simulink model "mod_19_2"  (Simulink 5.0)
settings: Solver=ode1  StartTime=0.0  StopTime=200  FixedStep=0.002  MaxStep=0.01  MinStep=0.0001  RelTol=1e-3
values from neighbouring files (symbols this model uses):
  Acp = 5.249    [dados_19_2.m]
  Apr = 5.249    [dados_19_2.m]
  CA0 = 12.815    [dados_19_2.m]
  CB0 = 0    [dados_19_2.m]
  cp = 0.12    [dados_19_2.m]
  cPa = 1.0    (= 1)    [dados_19_2.m]
  cPr = 1.0    (= 1)    [dados_19_2.m]
  Cva = 100    [dados_19_2.m]
  Cvv = 1.65    [dados_19_2.m]
  dPa = 1.406    [dados_19_2.m]
  G = 0.99803    [dados_19_2.m]
  hv_tab = [2706.3 2708.5 2710.6 2712.6 2714.5 2716.4 2718.2 2719.9 2721.5 2723.1 2724.7            2726.1 2727.6 2729.0 2730.0 2731.6]*0.2388459    [dados_19_2.m]
  k10 = 729.55    [dados_19_2.m]
  k20 = 6567.6    [dados_19_2.m]
  Kc = 2    [dados_19_2.m]
  Km = (Tmed_max-Tmed_min)/(Tmax-Tmin)    (= 0.109090909091)    [dados_19_2.m]
  Kva = 0.014276    [dados_19_2.m]
  Kvv = 6.4516    [dados_19_2.m]
  Lambda1 = 22222    [dados_19_2.m]
  Lambda2 = 27778    [dados_19_2.m]
  mcbarra = 7    [dados_19_2.m]
  Pv0 = 2.419    [dados_19_2.m]
  Pv_alim = 2.461    [dados_19_2.m]
  Pv_tab = [   2.0    2.1    2.2    2.3    2.4    2.5    2.6    2.7    2.8    2.9    3.0               3.1    3.2    3.3    3.4    3.5]*1.019716    [dados_19_2.m]
  R = 1.9858    [dados_19_2.m]
  rampa = 0.005    [dados_19_2.m]
  rho = 800.92    [dados_19_2.m]
  rhoa = 997.048    [dados_19_2.m]
  rhop = 8201.5    [dados_19_2.m]
  rhov_tab = [1/0.8854 1/0.8459 1/0.8098 1/0.7768 1/0.7465 1/0.7184 1/0.6925 1/0.6684 1/0.6460            1/0.6251 1/0.6056 1/0.5872 1/0.5700 1/0.5538 1/0.5385 1/0.5240]    [dados_19_2.m]
  T0 = 25    [dados_19_2.m]
  Tae = 25    [dados_19_2.m]
  talm = 4/60    (= 0.0666666666667)    [dados_19_2.m]
  Tlim = 93    [dados_19_2.m]
  Tmed0 = Km*(T0-Tmin)+Tmed_min    (= 4.63636363636)    [dados_19_2.m]
  Tmed_max = 15    [dados_19_2.m]
  Tmed_min = 3    [dados_19_2.m]
  Tmin = 10    [dados_19_2.m]
  Tp0 = 25    [dados_19_2.m]
  Tref0 = 12.6    [dados_19_2.m]
  Tv_tab = [120.23 121.78 123.27 124.71 126.09 127.43 128.73 129.98 131.20 132.39 133.54            134.66 135.75 136.82 137.86 138.87]    [dados_19_2.m]
  Uap = 32.550    (= 32.55)    [dados_19_2.m]
  Upr = 13.020    (= 13.02)    [dados_19_2.m]
  Uvp = 81.374    [dados_19_2.m]
  V = 1.2035    [dados_19_2.m]
  Vcam = 0.5332    [dados_19_2.m]
  Vp = 0.2667    [dados_19_2.m]
  xT = 0.75    [dados_19_2.m]
libraries: simulink_extras x1

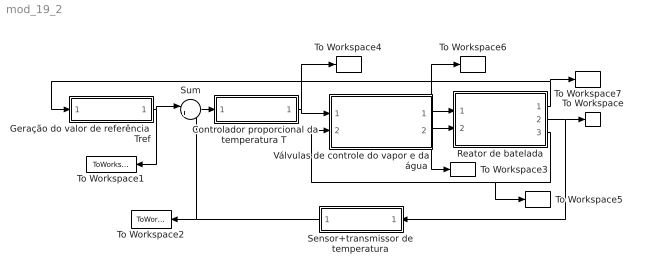
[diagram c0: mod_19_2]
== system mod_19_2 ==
  "Controlador proporcional da temperatura T " : Subsystem
  Geração do valor de referência Tref : Subsystem
  Reator de batelada : Subsystem
  Sensor+transmissor de temperatura : Subsystem  Orientation=left
  Sum : Sum  Inputs=|+-
  To Workspace : ToWorkspace  VariableName=T  SampleTime=-1  SaveFormat=Array
  To Workspace1 : ToWorkspace  VariableName=Tref_psi  SampleTime=-1  SaveFormat=Array
  To Workspace2 : ToWorkspace  VariableName=Tmed  SampleTime=-1  SaveFormat=Array
  To Workspace3 : ToWorkspace  VariableName=Wv  SampleTime=-1  SaveFormat=Array
  To Workspace4 : ToWorkspace  VariableName=mc  SampleTime=-1  SaveFormat=Array
  To Workspace5 : ToWorkspace  VariableName=Pv  SampleTime=-1  SaveFormat=Array
  To Workspace6 : ToWorkspace  VariableName=Qa  SampleTime=-1  SaveFormat=Array
  To Workspace7 : ToWorkspace  VariableName=Chav  SampleTime=-1  SaveFormat=Array
  "Válvulas de controle do vapor e da água " : Subsystem
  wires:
  Reator de batelada/1(Chav) -> Geração do valor de referência Tref/1(Chav), To Workspace7/1
  "Válvulas de controle do vapor e da água "/1(Qa) -> To Workspace6/1, Reator de batelada/1(Qa)
  "Controlador proporcional da temperatura T "/1(mc) -> To Workspace4/1, "Válvulas de controle do vapor e da água "/1(mc)
  Sum/1 -> "Controlador proporcional da temperatura T "/1(ec)
  Geração do valor de referência Tref/1(Tref_psi) -> Sum/1, To Workspace1/1
  Sensor+transmissor de temperatura/1(Tmed) -> Sum/2, To Workspace2/1
  Reator de batelada/2(T) -> To Workspace/1, Sensor+transmissor de temperatura/1(T)
  Reator de batelada/3(Pv) -> "Válvulas de controle do vapor e da água "/2(Pv), To Workspace5/1
  "Válvulas de controle do vapor e da água "/2(Wv) -> To Workspace3/1, Reator de batelada/2(Wv)

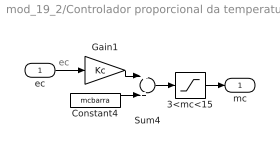
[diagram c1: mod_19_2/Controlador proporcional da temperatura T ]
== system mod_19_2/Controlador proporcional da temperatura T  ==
  note: ec
  ec : Inport
  3<mc<15 : Saturate  UpperLimit=15  LowerLimit=3
  Constant4 : Constant  Value=mcbarra
  Gain1 : Gain  Gain=Kc
  Sum4 : Sum  Inputs=2
  mc : Outport
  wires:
  ec/1 -> Gain1/1
  Gain1/1 -> Sum4/1
  Constant4/1 -> Sum4/2
  Sum4/1 -> 3<mc<15/1
  3<mc<15/1 -> mc/1

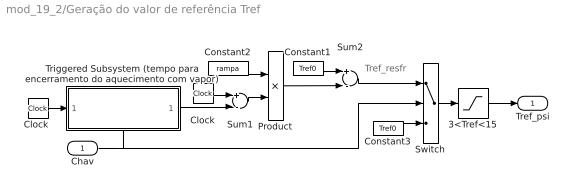
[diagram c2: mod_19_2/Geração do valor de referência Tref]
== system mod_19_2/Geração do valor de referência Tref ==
  note: Tref_resfr
  Chav : Inport
  3<Tref<15 : Saturate  UpperLimit=Tmed_max  LowerLimit=Tmed_min
  Clock : Clock
  "Clock " : Clock
  Constant1 : Constant  Value=Tref0
  Constant2 : Constant  Value=rampa
  Constant3 : Constant  Value=Tref0
  Product : Product
  Sum1 : Sum  Inputs=+-
  Sum2 : Sum  Inputs=+-
  Switch : Switch  Threshold=0.5
  Triggered Subsystem (tempo para encerramento do aquecimento com vapor) : Subsystem  TreatAsAtomicUnit=on
  Tref_psi : Outport
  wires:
  Triggered Subsystem (tempo para encerramento do aquecimento com vapor)/1(t_inicio_resfr) -> Sum1/2
  Constant3/1 -> Switch/3
  Switch/1 -> 3<Tref<15/1
  Sum2/1 -> Switch/1
  "Clock "/1 -> Triggered Subsystem (tempo para encerramento do aquecimento com vapor)/1(tempo)
  Chav/1 -> Triggered Subsystem (tempo para encerramento do aquecimento com vapor)/Trigger, Switch/2
  Clock/1 -> Sum1/1
  Sum1/1 -> Product/2
  Constant2/1 -> Product/1
  Constant1/1 -> Sum2/1
  Product/1 -> Sum2/2
  3<Tref<15/1 -> Tref_psi/1

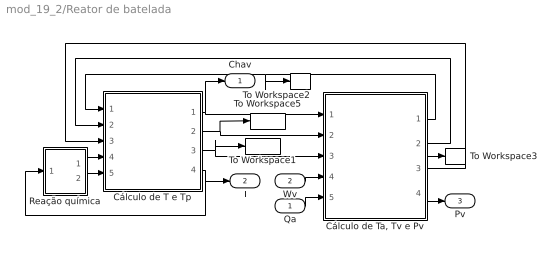
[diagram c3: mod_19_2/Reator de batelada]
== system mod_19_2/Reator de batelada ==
  Qa : Inport
  Wv : Inport  Port=2
  Cálculo de T e Tp : Subsystem
  "Cálculo de Ta, Tv e Pv" : Subsystem
  Reação química : Subsystem
  To Workspace1 : ToWorkspace  VariableName=qcp_r  SampleTime=-1  SaveFormat=Array
  To Workspace2 : ToWorkspace  VariableName=Tv  SampleTime=-1  SaveFormat=Array
  To Workspace3 : ToWorkspace  VariableName=Ta  SampleTime=-1  SaveFormat=Array
  To Workspace5 : ToWorkspace  VariableName=qcp_a  SampleTime=-1  SaveFormat=Array
  Chav : Outport
  T : Outport  Port=2
  Pv : Outport  Port=3
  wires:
  Qa/1 -> "Cálculo de Ta, Tv e Pv"/5(Qa)
  Wv/1 -> "Cálculo de Ta, Tv e Pv"/4(Wv)
  "Cálculo de Ta, Tv e Pv"/4(Pv) -> Pv/1
  Cálculo de T e Tp/2(qcp_aquec) -> "Cálculo de Ta, Tv e Pv"/2(qcp_aquec), To Workspace5/1
  "Cálculo de Ta, Tv e Pv"/1(Tv) -> Cálculo de T e Tp/1(Tv), To Workspace2/1
  Cálculo de T e Tp/1(Chav) -> "Cálculo de Ta, Tv e Pv"/1(Chav), Chav/1
  Cálculo de T e Tp/4(T) -> Reação química/1(T), T/1
  Reação química/2(q2) -> Cálculo de T e Tp/5(q2)
  Reação química/1(q1) -> Cálculo de T e Tp/4(q1)
  "Cálculo de Ta, Tv e Pv"/2(Ta) -> Cálculo de T e Tp/2(Ta), To Workspace3/1
  "Cálculo de Ta, Tv e Pv"/3(Va,cam) -> Cálculo de T e Tp/3(Va,cam)
  Cálculo de T e Tp/3(qcp_resfr) -> "Cálculo de Ta, Tv e Pv"/3(qcp_resfr), To Workspace1/1

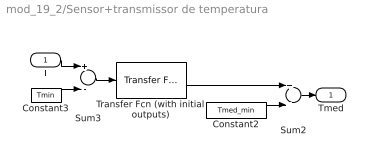
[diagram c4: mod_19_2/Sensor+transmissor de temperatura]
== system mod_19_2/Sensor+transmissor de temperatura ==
  T : Inport
  Constant2 : Constant  Value=Tmed_min
  Constant3 : Constant  Value=Tmin
  Sum2 : Sum  Inputs=2
  Sum3 : Sum  Inputs=+-
  Transfer Fcn (with initial outputs) : simulink_extras/Additional Linear/Transfer Fcn (with initial outputs)  N=[Km]  D="[talm  1]"  Y0=Tmed0-Tmed_min  U0=0
  Tmed : Outport
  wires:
  T/1 -> Sum3/1
  Sum2/1 -> Tmed/1
  Constant3/1 -> Sum3/2
  Sum3/1 -> Transfer Fcn (with initial outputs)/1
  Transfer Fcn (with initial outputs)/1 -> Sum2/1
  Constant2/1 -> Sum2/2

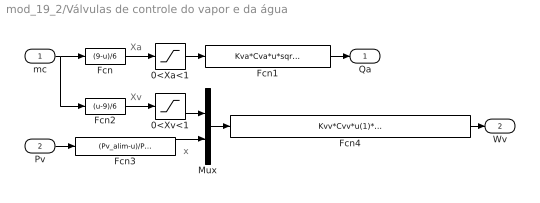
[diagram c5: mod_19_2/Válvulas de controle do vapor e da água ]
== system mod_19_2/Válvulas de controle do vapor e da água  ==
  note: Xa
  note: Xv
  note: x
  mc : Inport
  Pv : Inport  Port=2
  0<Xa<1 : Saturate  UpperLimit=1  LowerLimit=0
  0<Xv<1 : Saturate  UpperLimit=1  LowerLimit=0
  Fcn : Fcn  Expr=(9-u)/6
  Fcn1 : Fcn  Expr=Kva*Cva*u*sqrt(dPa/G)
  Fcn2 : Fcn  Expr=(u-9)/6
  Fcn3 : Fcn  Expr=(Pv_alim-u)/Pv_alim
  Fcn4 : Fcn  Expr=Kvv*Cvv*u(1)*Pv_alim*(3-u(2)/xT)*sqrt(u(2))
  Mux : Mux  Inputs=2
  Qa : Outport
  Wv : Outport  Port=2
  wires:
  mc/1 -> Fcn/1, Fcn2/1
  Fcn/1 -> 0<Xa<1/1
  0<Xa<1/1 -> Fcn1/1
  Fcn2/1 -> 0<Xv<1/1
  0<Xv<1/1 -> Mux/1
  Fcn1/1 -> Qa/1
  Pv/1 -> Fcn3/1
  Mux/1 -> Fcn4/1
  Fcn4/1 -> Wv/1
  Fcn3/1 -> Mux/2

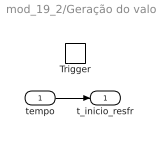
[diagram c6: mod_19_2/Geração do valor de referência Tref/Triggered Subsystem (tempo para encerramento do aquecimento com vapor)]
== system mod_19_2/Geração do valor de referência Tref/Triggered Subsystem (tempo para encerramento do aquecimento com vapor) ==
  tempo : Inport
  Trigger : TriggerPort
  t_inicio_resfr : Outport
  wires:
  tempo/1 -> t_inicio_resfr/1

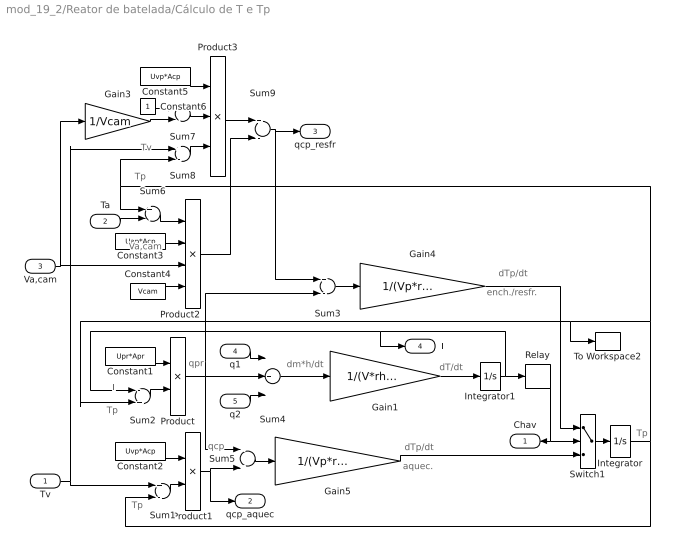
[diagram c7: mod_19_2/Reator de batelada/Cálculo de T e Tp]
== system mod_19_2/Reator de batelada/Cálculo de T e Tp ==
  note: Tp
  note: dTp/dt
  note: T
  note: dT/dt
  note: dm*h/dt
  note: qcp
  note: Tp
  note: qpr
  note: Tp
  note: aquec.
  note: Va,cam
  note: Tp
  note: Tv
  note: dTp/dt
  note: ench./resfr.
  Tv : Inport
  Ta : Inport  Port=2
  Va,cam : Inport  Port=3
  q1 : Inport  Port=4
  q2 : Inport  Port=5
  Constant1 : Constant  Value=Upr*Apr
  Constant2 : Constant  Value=Uvp*Acp
  Constant3 : Constant  Value=Uap*Acp
  Constant4 : Constant  Value=Vcam
  Constant5 : Constant  Value=Uvp*Acp
  Constant6 : Constant
  Gain1 : Gain  Gain=1/(V*rho*cPr)
  Gain3 : Gain  Gain=1/Vcam
  Gain4 : Gain  Gain=1/(Vp*rhop*cp)
  Gain5 : Gain  Gain=1/(Vp*rhop*cp)
  Integrator : Integrator  InitialCondition=Tp0
  Integrator1 : Integrator  InitialCondition=T0
  Product : Product
  Product1 : Product
  Product2 : Product  Inputs=***/
  Product3 : Product  Inputs=3
  Relay : Relay  OnSwitchValue=Tlim  OffSwitchValue=T0
  Sum{1,3,6..9} (6 alike) : Sum  Inputs=+-
  Sum2 : Sum  Inputs=-+
  Sum4 : Sum  Inputs=3
  Sum5 : Sum  Inputs=-+
  Switch1 : Switch  Threshold=0.5
  To Workspace2 : ToWorkspace  VariableName=Tp  SampleTime=-1  SaveFormat=Array
  Chav : Outport  Orientation=left
  qcp_aquec : Outport  Port=2
  qcp_resfr : Outport  Port=3
  T : Outport  Port=4
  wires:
  Integrator1/1 -> Relay/1, Sum2/1, T/1
  Integrator/1 -> Sum1/2, Sum2/2, To Workspace2/1, Sum6/1, Sum8/2
  Sum1/1 -> Product1/2
  Gain1/1 -> Integrator1/1
  Sum4/1 -> Gain1/1
  q1/1 -> Sum4/1
  q2/1 -> Sum4/3
  Product1/1 -> qcp_aquec/1, Sum5/2
  Tv/1 -> Sum1/1, Sum8/1
  Product/1 -> Sum5/1, Sum4/2, Sum3/2
  Constant1/1 -> Product/1
  Sum2/1 -> Product/2
  Constant2/1 -> Product1/1
  Constant3/1 -> Product2/2
  Va,cam/1 -> Product2/3, Gain3/1
  Constant4/1 -> Product2/4
  Ta/1 -> Sum6/2
  Sum6/1 -> Product2/1
  Gain3/1 -> Sum7/2
  Constant6/1 -> Sum7/1
  Sum7/1 -> Product3/2
  Constant5/1 -> Product3/1
  Sum8/1 -> Product3/3
  Sum3/1 -> Gain4/1
  Sum5/1 -> Gain5/1
  Switch1/1 -> Integrator/1
  Relay/1 -> Switch1/2, Chav/1
  Gain4/1 -> Switch1/1
  Gain5/1 -> Switch1/3
  Product3/1 -> Sum9/1
  Product2/1 -> Sum9/2
  Sum9/1 -> qcp_resfr/1, Sum3/1

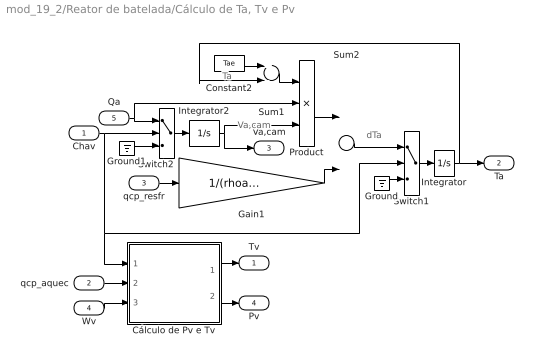
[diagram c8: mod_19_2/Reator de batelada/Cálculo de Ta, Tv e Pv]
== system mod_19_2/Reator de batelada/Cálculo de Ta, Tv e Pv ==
  note: dTa
  note: Ta
  note: Va,cam
  Chav : Inport
  qcp_aquec : Inport  Port=2
  qcp_resfr : Inport  Port=3
  Wv : Inport  Port=4
  Qa : Inport  Port=5
  Constant2 : Constant  Value=Tae
  Cálculo de Pv e Tv : Subsystem
  Gain1 : Gain  Gain=1/(rhoa*Vcam*cPa)
  Ground : Ground
  Ground1 : Ground
  Integrator : Integrator  InitialCondition=Tae
  Integrator2 : Integrator  InitialCondition=0.0001  LimitOutput=on  UpperSaturationLimit=Vcam  LowerSaturationLimit=0.0001
  Product : Product  Inputs=**/
  Sum1 : Sum  Inputs=+-
  Sum2 : Sum  Inputs=+-
  Switch1 : Switch  Threshold=0.5
  Switch2 : Switch  Threshold=0.5
  Tv : Outport
  Ta : Outport  Port=2
  Va,cam : Outport  Port=3
  Pv : Outport  Port=4
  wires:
  Integrator/1 -> Ta/1, Sum1/2
  Wv/1 -> Cálculo de Pv e Tv/3(Wv)
  Cálculo de Pv e Tv/1(Tv) -> Tv/1
  Cálculo de Pv e Tv/2(Pv) -> Pv/1
  Gain1/1 -> Sum2/2
  Qa/1 -> Switch2/1, Product/2
  Ground1/1 -> Switch2/3
  Switch2/1 -> Integrator2/1
  Integrator2/1 -> Product/3, Va,cam/1
  Sum2/1 -> Switch1/1
  Switch1/1 -> Integrator/1
  Ground/1 -> Switch1/3
  Constant2/1 -> Sum1/1
  Product/1 -> Sum2/1
  Sum1/1 -> Product/1
  Chav/1 -> Switch2/2, Switch1/2, Cálculo de Pv e Tv/1(Chav)
  qcp_resfr/1 -> Gain1/1
  qcp_aquec/1 -> Cálculo de Pv e Tv/2(qcp_aquec)

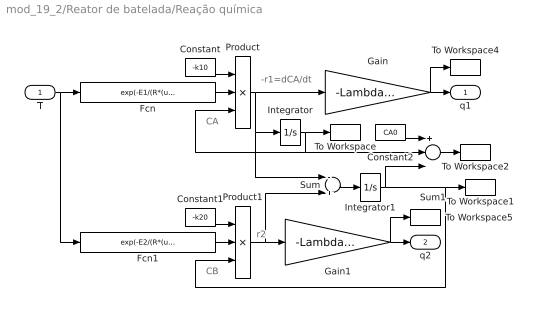
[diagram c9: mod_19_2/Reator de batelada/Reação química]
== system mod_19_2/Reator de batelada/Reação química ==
  note: r2
  note: CB
  note: -r1=dCA/dt
  note: CA
  T : Inport
  Constant : Constant  Value=-k10
  Constant1 : Constant  Value=-k20
  Constant2 : Constant  Value=CA0
  Fcn : Fcn  Expr=exp(-E1/(R*(u+273.15)))
  Fcn1 : Fcn  Expr=exp(-E2/(R*(u+273.15)))
  Gain : Gain  Gain=-Lambda1*V
  Gain1 : Gain  Gain=-Lambda2*V
  Integrator : Integrator  InitialCondition=CA0
  Integrator1 : Integrator  InitialCondition=CB0
  Product : Product  Inputs=3
  Product1 : Product  Inputs=3
  Sum : Sum  Inputs=-+
  Sum1 : Sum  Inputs=+--
  To Workspace : ToWorkspace  VariableName=CA  SampleTime=-1  SaveFormat=Array
  To Workspace1 : ToWorkspace  VariableName=CB  SampleTime=-1  SaveFormat=Array
  To Workspace2 : ToWorkspace  VariableName=CC  SampleTime=-1  SaveFormat=Array
  To Workspace4 : ToWorkspace  VariableName=q1  SampleTime=-1  SaveFormat=Array
  To Workspace5 : ToWorkspace  VariableName=q2  SampleTime=-1  SaveFormat=Array
  q1 : Outport
  q2 : Outport  Port=2
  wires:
  Constant1/1 -> Product1/1
  Sum1/1 -> To Workspace2/1
  Constant2/1 -> Sum1/1
  Sum/1 -> Integrator1/1
  Integrator1/1 -> Product1/3, To Workspace1/1, Sum1/3
  Integrator/1 -> Product/3, Sum1/2, To Workspace/1
  Gain1/1 -> q2/1, To Workspace5/1
  Gain/1 -> q1/1, To Workspace4/1
  Product1/1 -> Sum/2, Gain1/1
  Fcn1/1 -> Product1/2
  Product/1 -> Sum/1, Integrator/1, Gain/1
  Constant/1 -> Product/1
  Fcn/1 -> Product/2
  T/1 -> Fcn1/1, Fcn/1

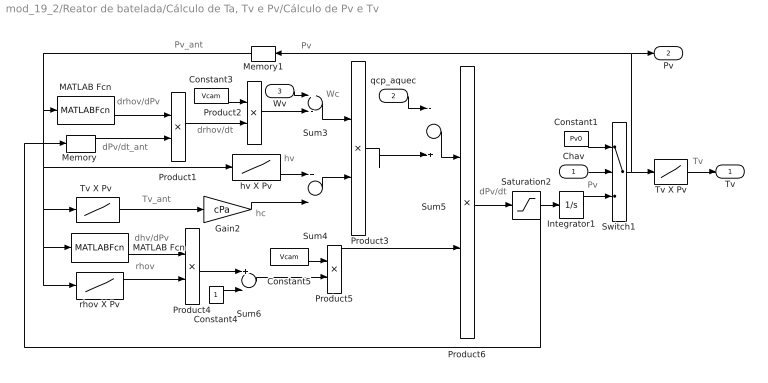
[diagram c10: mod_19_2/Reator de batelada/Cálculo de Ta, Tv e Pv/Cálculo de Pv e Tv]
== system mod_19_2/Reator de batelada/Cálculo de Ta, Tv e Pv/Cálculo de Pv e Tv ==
  note: Tv
  note: Pv
  note: dPv/dt
  note: rhov
  note: Pv
  note: dhv/dPv
  note: hc
  note: Tv_ant
  note: hv
  note: drhov/dt
  note: dPv/dt_ant
  note: drhov/dPv
  note: Pv_ant
  note: Wc
  Chav : Inport
  qcp_aquec : Inport  Port=2
  Wv : Inport  Port=3
  Constant1 : Constant  Value=Pv0
  Constant3 : Constant  Value=Vcam
  Constant4 : Constant
  Constant5 : Constant  Value=Vcam
  Gain2 : Gain  Gain=cPa
  Integrator1 : Integrator  InitialCondition=Pv0  LimitOutput=on  UpperSaturationLimit=Pv_alim  LowerSaturationLimit=0
  MATLAB Fcn : MATLABFcn  MATLABFcn=drhov_dPv
  "MATLAB Fcn " : MATLABFcn  MATLABFcn=dhv_dPv
  "Memory " : Memory
  Memory1 : Memory  Orientation=left  X0=Pv0
  Product{1..5} (5 alike) : Product
  Product6 : Product  Inputs=*/
  Saturation2 : Saturate  UpperLimit=0.005  LowerLimit=-0.005
  Sum3 : Sum  Inputs=+-
  Sum4 : Sum  Inputs=+-
  Sum5 : Sum  Inputs=-+
  Sum6 : Sum  Inputs=+-
  Switch1 : Switch  Threshold=0.5
  Tv X Pv : Lookup  InputValues=Pv_tab  OutputValues=Tv_tab
  "Tv X Pv " : Lookup  InputValues=Pv_tab  OutputValues=Tv_tab
  hv X Pv : Lookup  InputValues=Pv_tab  OutputValues=hv_tab
  rhov X Pv : Lookup  InputValues=Pv_tab  OutputValues=rhov_tab
  Tv : Outport
  Pv : Outport  Port=2
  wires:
  qcp_aquec/1 -> Sum5/1
  Memory1/1 -> "Tv X Pv "/1, "MATLAB Fcn "/1, rhov X Pv/1, hv X Pv/1, MATLAB Fcn/1
  Saturation2/1 -> Integrator1/1, "Memory "/1
  Product6/1 -> Saturation2/1
  Sum5/1 -> Product6/1
  Product5/1 -> Product6/2
  Constant5/1 -> Product5/1
  Sum6/1 -> Product5/2
  Constant4/1 -> Sum6/2
  Product4/1 -> Sum6/1
  rhov X Pv/1 -> Product4/2
  "MATLAB Fcn "/1 -> Product4/1
  Product3/1 -> Sum5/2
  Sum4/1 -> Product3/2
  Gain2/1 -> Sum4/2
  "Tv X Pv "/1 -> Gain2/1
  hv X Pv/1 -> Sum4/1
  Product2/1 -> Sum3/2
  Constant3/1 -> Product2/1
  Sum3/1 -> Product3/1
  Product1/1 -> Product2/2
  "Memory "/1 -> Product1/2
  MATLAB Fcn/1 -> Product1/1
  Wv/1 -> Sum3/1
  Chav/1 -> Switch1/2
  Switch1/1 -> Tv X Pv/1, Memory1/1, Pv/1
  Integrator1/1 -> Switch1/3
  Tv X Pv/1 -> Tv/1
  Constant1/1 -> Switch1/1
